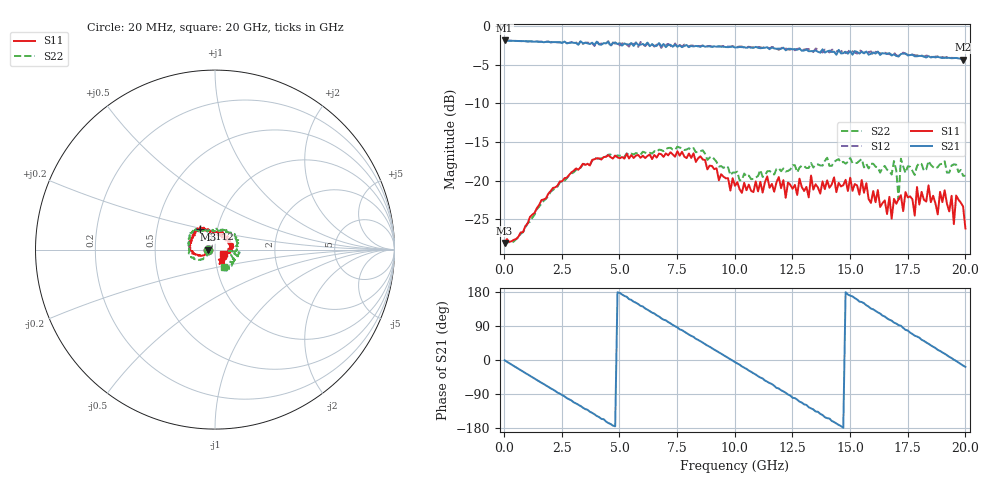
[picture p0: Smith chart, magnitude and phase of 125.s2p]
!Agilent Technologies,N5230A,US43500223,A.07.50.48
!Agilent N5230A: A.07.50.48
!Date: Saturday, September 19, 2015 18:55:31
!Correction: S11(Full 2 Port(1,2))
!S21(Full 2 Port(1,2))
!S12(Full 2 Port(1,2))
!S22(Full 2 Port(1,2))
!S2P File: Measurements: S11, S21, S12, S22:
# Hz S  RI  R 50
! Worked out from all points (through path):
!   201 points, 20 MHz to 20 GHz, reference 50 ohm
!   highest |S21| = -1.82 dB at 20 MHz (marker M1); lowest = -4.3 dB at 19.9 GHz (marker M2)
!   group delay of S21, straight-line fit = 102 ps
!   lowest |S11| = -28.1 dB at 20 MHz (marker M3), VSWR 1.08, Z = 46.2 + j0.0154 ohm
!   |S11| at or under -10 dB: start of sweep to end of sweep
!   |S22| runs from -28.5 to -15.6 dB; largest |S21 - S12| = 0.07
!   S11 on the Smith chart (normalised r, x): 20 MHz: 0.92, +0.00; 8.112 GHz: 0.83, +0.19; 20 GHz: 1.09, -0.05
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2e7  -0.0393 0.000166  0.8106 -0.0109  0.8096 -0.012  -0.0375 -0.000178
1.9181e9  -0.0743 -0.0352  0.2607 -0.7538  0.264 -0.7512  -0.063 -0.0491
3.4166e9  -0.1265 -0.0224  -0.4535 -0.6298  -0.4544 -0.6215  -0.1165 -0.0521
4.9151e9  -0.1375 0.0335  -0.768 0.0172  -0.7878 0.0256  -0.1454 -0.00266
6.7133e9  -0.1154 0.095  -0.3258 0.7082  -0.3376 0.7031  -0.147 0.0596
8.1119e9  -0.0814 0.1141  0.3308 0.6691  0.3091 0.6861  -0.1255 0.0969
1.001e10  -0.00504 0.0921  0.7264 -0.0722  0.7336 -0.0459  -0.0327 0.1076
1.17083e10  0.0293 0.0793  0.2695 -0.6672  0.2984 -0.6724  0.0345 0.1037
1.34066e10  0.0685 0.0541  -0.4497 -0.5263  -0.4146 -0.5425  0.0915 0.0797
1.5005e10  0.1029 0.0173  -0.6798 0.1233  -0.7034 0.0786  0.1295 0.0538
1.67033e10  0.0693 -0.0366  -0.1886 0.6445  -0.2226 0.6209  0.1128 -0.0196
1.68032e10  0.0519 -0.0225  -0.1546 0.6286  -0.1776 0.6355  0.1069 -0.0226
1.69031e10  0.0571 -0.0502  -0.0987 0.6516  -0.1387 0.6622  0.1287 -0.0367
1.71029e10  0.0336 -0.0679  -0.0226 0.6368  -0.0687 0.6409  0.0752 -0.00609
1.72028e10  0.0484 -0.064  -0.00608 0.662  -0.0401 0.6621  0.1376 -0.0161
1.78022e10  0.0208 -0.0555  0.2788 0.5759  0.2504 0.6002  0.0854 -0.0673
1.86014e10  0.0271 -0.0749  0.5201 0.3644  0.4945 0.3927  0.0747 -0.0967
1.94006e10  0.0599 -0.0523  0.619 0.0549  0.6185 0.0892  0.0585 -0.1106
1.95005e10  0.0424 -0.0304  0.6228 0.00931  0.6217 0.0438  0.0638 -0.1102
1.96004e10  0.063 -0.0492  0.6237 -0.0285  0.624 0.00249  0.0518 -0.1156
1.99001e10  0.0551 -0.0398  0.589 -0.1547  0.6031 -0.1219  0.0383 -0.1002
2e10  0.0431 -0.0229  0.5836 -0.191  0.5949 -0.1552  0.0504 -0.0946
